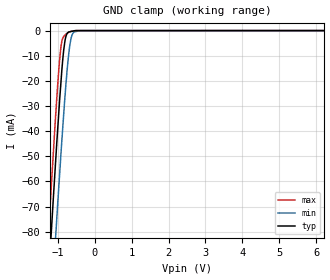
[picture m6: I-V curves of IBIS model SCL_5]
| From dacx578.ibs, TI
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|   SCL Model 5V MODEL
[Model] SCL_5
Model_type   Input
Vinl = 1.5
Vinh = 3.5
|   typ   min   max
|   (Nom PVT)   (Fast PVT)  (Slow PVT)
C_comp   1.0142160e-12   8.6172550e-13   1.1527990e-12
|Where nom PVT is Nom process, 5.0V, 27C
|Fast PVT is Strong Process, 5.5V, -40C
|Slow PVT is Weak Process,   4.5V, 125C
[Voltage Range]   5   4.5   5.5
[Temperature Range]   27   125   -40
|Junction temperatures are used for [Temperature Range]
[Power Clamp Reference]   5   4.5   5.5
[GND Clamp Reference]   0   0   0
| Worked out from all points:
|   GND clamp passes 1 mA (typ) near -0.73 V on its own axis
[GND Clamp]
|   Voltage   I(typ)   I(min)   I(max)
-5V       -1.085A    -1.1A      -1.078A
-1.243V   -97.38mA   -127.3mA   -79.5mA
-1.158V   -76.62mA   -106.5mA   -58.42mA
-1.059V   -52.82mA   -82.92mA   -34.65mA
-1.028V   -45.56mA   -75.63mA   -27.81mA
-919.1mV  -22.1mA    -50.8mA    -7.416mA
-862.5mV  -11.56mA   -38.64mA   -3.041mA
-799.1mV  -3.757mA   -25.65mA   -1.729mA
-705.7mV  -590.8uA   -10mA      -720.7uA
-611.1mV  -288.3uA   -1.778mA   -198uA
-399.7mV  -14.36uA   -11.64uA   -14.35uA
9.985V    0A         0A         0A
[POWER Clamp]
|   SCR cell for ESD function. Effects occurr above VDD x 2
|   Voltage   I(typ)   I(min)   I(max)
-5V       0A         0A         0A
0V        0A         0A         0A
10V       0A         0A         0A
